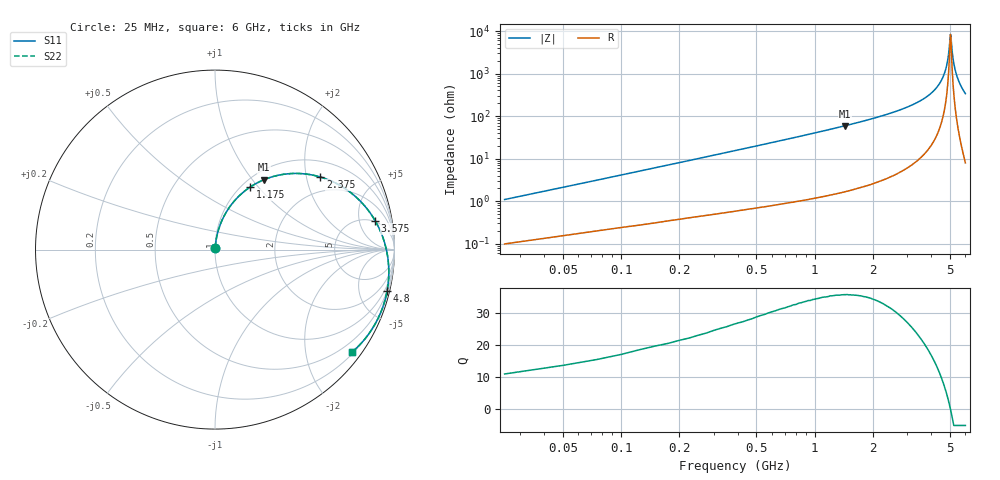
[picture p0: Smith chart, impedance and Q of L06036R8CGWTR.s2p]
!	AVX Thin Film Operation
!	Date:	March	2003
!	Description: Accu-L® Series Thin Film SMD RF Inductors
!	Part Number: L06036R8CGWTR
!	25MHz-6GHz
!	Serial	Measurements
#	mhz	S	db	R	50
!	S11	S11	S21	S21	S12	S12	S22	S22
!	dB	Phase	dB	Phase	dB	Phase	dB	Phase
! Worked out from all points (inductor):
!   240 points, 25 MHz to 6 GHz, reference 50 ohm
!   read as one part in series: L = 6.59 nH near 50 MHz
!   highest Q = 35.7 at 1.425 GHz (marker M1), where L = 6.56 nH
!   self-resonance near 5.025 GHz
!   S11 on the Smith chart (normalised r, x): 25 MHz: 1.00, +0.02; 1.175 GHz: 1.09, +0.91; 2.375 GHz: 1.47, +2.42; 3.575 GHz: 4.76, +8.60; 4.8 GHz: 0.49, -8.33; 6 GHz: 0.24, -3.01
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25  -39.87 83.8  -0.01 -0.7  -0.01 -0.7  -39.87 83.8
50  -34.16 84.2  -0.01 -1.3  -0.01 -1.3  -34.16 84.2
100  -28.40 83.9  -0.03 -2.5  -0.03 -2.5  -28.40 83.9
175  -23.72 82.7  -0.05 -4.3  -0.05 -4.3  -23.72 82.7
275  -19.92 80.7  -0.08 -6.7  -0.08 -6.7  -19.92 80.7
575  -13.76 74.1  -0.25 -13.8  -0.25 -13.8  -13.76 74.1
1025  -9.04 64.0  -0.67 -24.1  -0.67 -24.1  -9.04 64.0
1175  -7.96 60.6  -0.86 -27.5  -0.86 -27.5  -7.96 60.6
1425  -6.48 55.1  -1.23 -33.1  -1.23 -33.1  -6.48 55.1
2025  -3.97 42.0  -2.41 -46.1  -2.41 -46.1  -3.97 42.0
2375  -2.94 34.6  -3.31 -53.4  -3.31 -53.4  -2.94 34.6
3025  -1.59 21.2  -5.51 -66.5  -5.51 -66.5  -1.59 21.2
3575  -0.85 10.2  -8.16 -77.0  -8.16 -77.0  -0.85 10.2
4025  -0.45 1.4  -11.31 -85.0  -11.31 -85.0  -0.45 1.4
4500  -0.20 -7.9  -16.82 -92.1  -16.82 -92.1  -0.20 -7.9
4800  -0.12 -13.6  -23.96 -91.9  -23.96 -91.9  -0.12 -13.6
4900  -0.11 -15.6  -28.63 -86.1  -28.63 -86.1  -0.11 -15.6
5025  -0.10 -18.0  -38.71 -22.7  -38.71 -22.7  -0.10 -18.0
5175  -0.11 -20.8  -27.72 54.2  -27.72 54.2  -0.11 -20.8
5325  -0.13 -23.7  -21.85 59.4  -21.85 59.4  -0.13 -23.7
5600  -0.20 -29.0  -16.23 58.1  -16.23 58.1  -0.20 -29.0
6000  -0.41 -36.6  -11.71 52.2  -11.71 52.2  -0.41 -36.6
